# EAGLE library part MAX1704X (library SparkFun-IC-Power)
MAX17043/MAX17044: Battery Fuel Guage (43 is 1cell, 44 is 2cell)
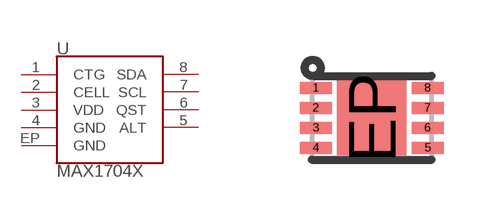
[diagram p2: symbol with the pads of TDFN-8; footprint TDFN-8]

Designator prefix U

## MAX1704X (PROD-ID: IC-10399)  [TDFN-8]
1  CTG
2  CELL
3  VDD
4  GND
5  ALT
6  QST
7  SCL
8  SDA
EP  GND

## Footprint TDFN-8 (pad centres in mm)
TDFN - 8pin, 2mmx3mm
smd 0.8 x 0.3: 1 -1.4,0.75; 2 -1.4,0.25; 3 -1.4,-0.25; 4 -1.4,-0.75; 5 1.4,-0.75; 6 1.4,-0.25; 7 1.4,0.25; 8 1.4,0.75
smd 1.73 x 1.88: EP 0,0

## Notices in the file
Licensing: Creative Commons ShareAlike 4.0 International - https://creativecommons.org/licenses/by-sa/4.0
